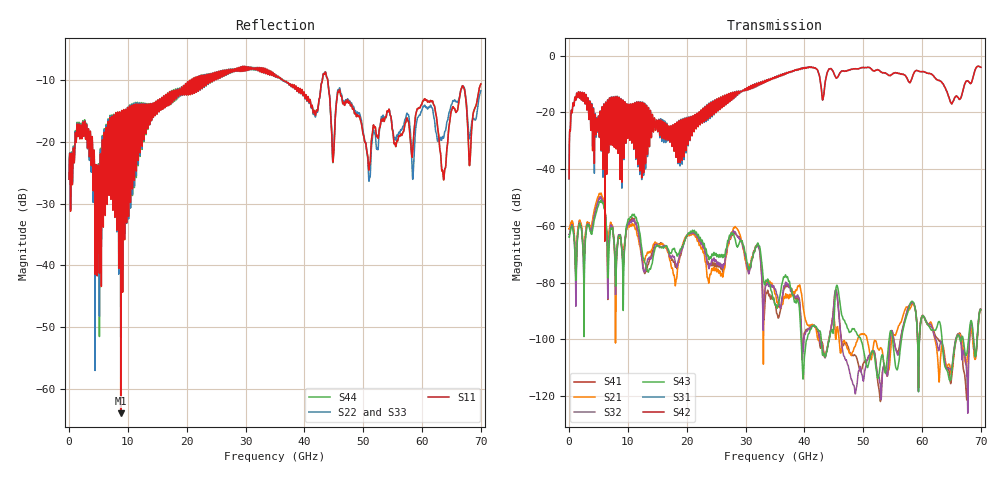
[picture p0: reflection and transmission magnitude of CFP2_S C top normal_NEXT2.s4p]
! AWR Design Environment (8415) Tue Jan 08 13:13:04 2019
! Document = 'CFP2 Channel_S'
! nPorts: 4, nXvals: 7001
# HZ S DB R 50
!Freq DBS11 AngS11 DBS12 AngS12 DBS13 AngS13 DBS14 AngS14
!	DBS21 AngS21 DBS22 AngS22 DBS23 AngS23 DBS24 AngS24
!	DBS31 AngS31 DBS32 AngS32 DBS33 AngS33 DBS34 AngS34
!	DBS41 AngS41 DBS42 AngS42 DBS43 AngS43 DBS44 AngS44
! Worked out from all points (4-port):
!   7000 points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, 10 MHz to 70 GHz, reference 50 ohm
!   strongest paths, dB at 10 MHz, 17.51 GHz, 35.01 GHz, 52.51 GHz, 70 GHz:
!     S42: -43.4, -31.9, -7.4, -5.0, -4.0
!     S31: -43.5, -31.2, -7.4, -5.0, -4.0
!     S43: -64.0, -68.6, -88.0, -113.8, -89.6
!     S32: -63.1, -70.6, -82.3, -112.6, -89.4
!     S21: -61.0, -74.9, -84.1, -103.3, -89.5
!     S41: -61.0, -71.8, -87.5, -115.6, -89.6
!   lowest |S11| = -63.9 dB at 8.78 GHz (marker M1), VSWR 1.00, Z = 50 + j0.058 ohm
!   |S11| at or under -10 dB: start of sweep to 20.78 GHz; 36.27 GHz to 43.07 GHz (6.797 GHz wide, 17.1 % of centre); 43.96 GHz to end of sweep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
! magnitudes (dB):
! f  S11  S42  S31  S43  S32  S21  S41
! 10 MHz  -26.1  -43.4  -43.5  -64.0  -63.1  -61.0  -61.0
! 1.34 GHz  -17.4  -13.2  -13.2  -68.0  -67.8  -66.4  -66.6
! 5.26 GHz  -23.9  -20.3  -20.5  -51.7  -50.3  -48.8  -50.0
! 8.78 GHz  -63.9  -15.8  -15.7  -64.1  -64.1  -64.6  -64.8
! 30.83 GHz  -8.0  -10.9  -10.9  -74.5  -75.0  -73.4  -74.9
! 63.66 GHz  -26.2  -10.2  -10.2  -106.6  -104.4  -103.1  -105.2
! 70 GHz  -10.7  -4.0  -4.0  -89.6  -89.4  -89.5  -89.6
